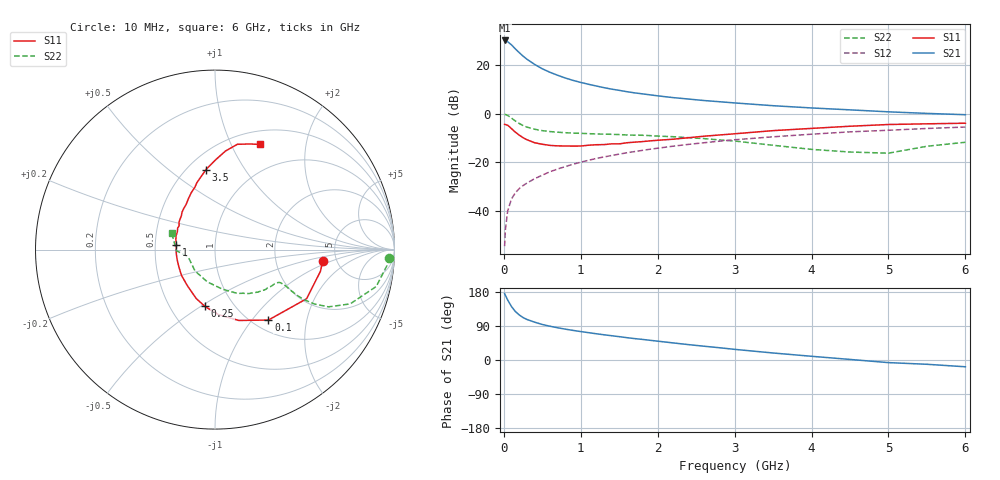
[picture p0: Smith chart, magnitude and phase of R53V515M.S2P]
! SIEMENS Small Signal Semiconductors
! BFR183
! Si NPN RF Bipolar Junction Transistor in SOT23
! VCE = 3.5 V  IC = 15 mA
! Common Emitter S-Parameters:  May  1996
# GHz  S  MA  R  50
!  f  S11  S21  S12  S22
! GHz  MAG  ANG  MAG  ANG  MAG  ANG  MAG  ANG
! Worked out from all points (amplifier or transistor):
!   36 points, 10 MHz to 6 GHz, reference 50 ohm
!   highest |S21| = 30.1 dB at 10 MHz (marker M1)
!   |S21| within 3 dB of that: start of sweep to 135.4 MHz
!   unconditionally stable (mu >= 1): 647.9 MHz to 2.43 GHz
!   at 250 MHz: K = 0.74, MSG = 26.6 dB, |S12| = -29.5 dB
!   at 1.4 GHz: K = 1.05, MAG = 12.3 dB, |S12| = -17.2 dB
!   at 6 GHz: K = 0.90, MSG = 2.5 dB, |S12| = -5.5 dB
!   S11 on the Smith chart (normalised r, x): 10 MHz: 3.89, -0.75; 100 MHz: 1.17, -1.21; 250 MHz: 0.74, -0.52; 1 GHz: 0.65, +0.04; 3.5 GHz: 0.61, +0.69; 6 GHz: 0.66, +1.30
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0.01  0.6037 -5.8  31.95 175.3  0.0019 89.8  0.9707 -2.6
0.02  0.5998 -11.6  31.58 170.7  0.0041 87.4  0.9617 -5.4
0.05  0.5792 -28.2  30.07 158.2  0.0101 76.7  0.9216 -12.9
0.1  0.4927 -52.8  25.89 140.9  0.0178 70.9  0.8113 -21.9
0.15  0.4166 -71.4  21.39 127.9  0.0238 67.4  0.7076 -26.8
0.2  0.3631 -86.9  17.97 118.9  0.0289 66.4  0.6299 -28.7
0.25  0.3212 -100.1  15.24 112.0  0.0334 65.7  0.5711 -29.3
0.3  0.292 -111.0  13.17 107.0  0.0376 66.3  0.5306 -29.2
0.4  0.2532 -127.5  10.29 99.9  0.0462 67.3  0.4795 -28.3
0.5  0.2356 -142.4  8.366 93.7  0.0547 68.7  0.4481 -27.4
0.6  0.2232 -154.3  7.085 89.1  0.0642 69.1  0.4292 -26.8
0.7  0.2183 -164.4  6.149 85.0  0.0732 69.5  0.4169 -26.9
0.8  0.217 -172.7  5.401 81.4  0.082 68.9  0.4066 -26.9
1  0.2165 172.5  4.386 75.0  0.101 68.6  0.3949 -27.8
1.1  0.2251 165.7  4.021 72.2  0.1103 68.0  0.3892 -29.0
1.3  0.2317 154.9  3.431 66.6  0.1292 66.7  0.3798 -30.8
1.6  0.253 142.4  2.83 58.9  0.1575 64.3  0.3657 -34.8
2.2  0.2989 122.5  2.141 45.1  0.215 58.6  0.3371 -44.6
3.5  0.449 96.4  1.459 18.5  0.3352 42.8  0.2245 -79.3
4.5  0.5525 83.9  1.199 1.5  0.4236 30.3  0.163 -133.0
5.5  0.6195 71.8  1.014 -11.3  0.4972 18.5  0.2141 -178.3
6  0.6374 66.8  0.953 -17.9  0.5318 10.9  0.259 158.9
